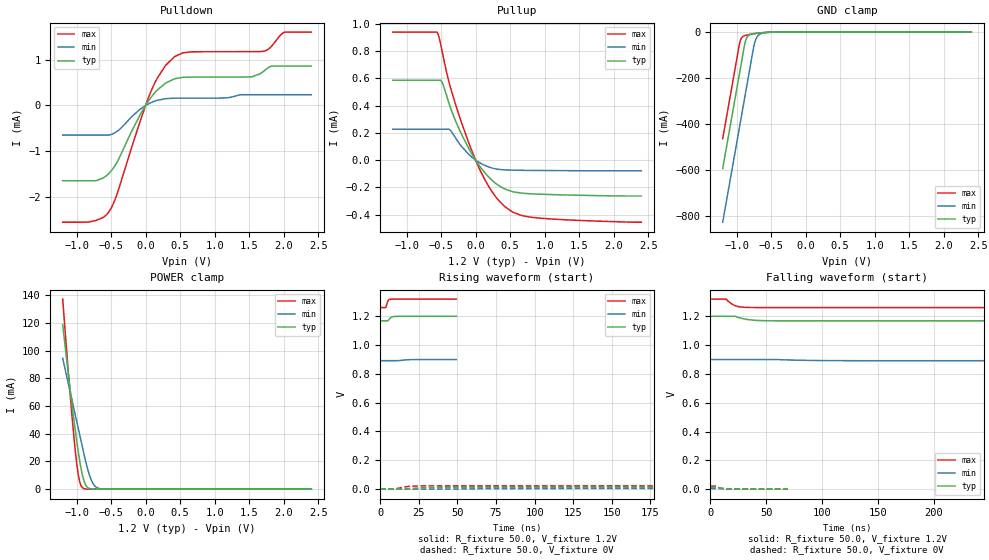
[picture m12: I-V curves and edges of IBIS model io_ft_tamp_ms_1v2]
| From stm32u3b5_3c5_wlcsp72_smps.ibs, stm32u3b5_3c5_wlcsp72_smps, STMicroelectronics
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[Model]   io_ft_tamp_ms_1v2
Model_type I/O
Polarity   Non-Inverting
Enable   Active-Low
| CAP_THRESHOLD on pad IOFT is "UDTCAPC" :
| Rising=30.0% of vddios   Falling=70.0% of vddios
| C_comp min and max val. don't necessarily correlate with the min and max pvt
| but are the smallest and greatest pad capacitance found.
| var   typ   min   max
C_comp   2.39258pF  2.36010pF  2.41953pF
|C_comp_pullup   1.38909pF  1.28768pF  1.47308pF
|C_comp_pulldown   1.00349pF  1.07242pF  946.45422fF
Vinl = 450.0mV
Vinh = 660.0mV
Vmeas = 600.0mV   | Reference voltage for timing measurements
Cref  = 50.0pF   | Timing specification test load capacitance value
Rref  = 1.0MOhm   | Timing specification test load resistance value
Vref  = 660.0mV   | Timing specification test load voltage
[Model Spec]
| TIME_THRESHOLD on pin ZIV11 is "CMOS" :
| Rising=50.0% of vdd   Falling=50.0% of vdd
Vinl 439.50000mV 331.50001mV 485.50000mV
Vinh 752.50000mV 552.50001mV 837.50000mV
| variable   typ   min   max
[Temperature Range] 25.0 130.0 -40.0
| variable   typ   min   max
[Voltage Range] 1.2V 900.0mV 1.32V
| variable   typ   min   max
[POWER Clamp Reference] 1.2V 900.0mV 1.32V
| variable   typ   min   max
[GND Clamp Reference] 0V 0V 0V
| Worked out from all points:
|   slope of the pulldown table from 0 to 0.18 V, typ, clamps not added: 514 ohm
|   slope of the pullup table from 0 to 0.18 V, typ, clamps not added: 1.52 kohm
|   GND clamp passes 1 mA (typ) near -0.53 V on its own axis
|   POWER clamp passes 1 mA (typ) near -0.83 V on its own axis
[POWER Clamp]
-1.2V     118.8mA    94.44mA    137.2mA
-1.09V    71.2mA     69.75mA    67.14mA
-1.02V    43.22mA    54.03mA    28.67mA
-990mV    32.26mA    47.3mA     15.78mA
-970mV    25.49mA    42.81mA    9.257mA
-940mV    16.45mA    36.08mA    3.257mA
-910mV    9.238mA    29.34mA    904.6uA
-860mV    2.387mA    18.53mA    87.46uA
-790mV    204.6uA    7.049mA    3.101uA
-730mV    21.91uA    2.041mA    176.4nA
-660mV    1.594uA    337.6uA    6.258nA
2.4V      0A         0A         0A
[GND Clamp]
-1.2V     -593.4mA   -826.9mA   -463.7mA
-960mV    -185.4mA   -418.9mA   -55.68mA
-940mV    -151.4mA   -384.9mA   -33.02mA
-880mV    -50.24mA   -282.9mA   -15.1mA
-850mV    -23.55mA   -231.9mA   -12.72mA
-810mV    -11.44mA   -163.9mA   -10.41mA
-740mV    -5.957mA   -49.45mA   -7.062mA
-710mV    -4.858mA   -24.97mA   -5.804mA
-670mV    -3.677mA   -10.87mA   -4.301mA
-590mV    -1.88mA    -3mA       -1.97mA
-390mV    -51.73uA   -182.4uA   -18.95uA
2.4V      708.1pA    117.2nA    245.1pA
| variable   typ   min   max
[Pullup Reference] 1.2V 900.0mV 1.32V
| variable   typ   min   max
[Pulldown Reference] 0V 0V 0V
[Pullup]
-1.2V     585.3uA    226.4uA    938.6uA
-550mV    585.3uA    226.4uA    931.1uA
-480mV    564.6uA    226.4uA    788uA
-360mV    379.5uA    215.3uA    526uA
-230mV    218.5uA    117.8uA    314.5uA
-80mV     67.47uA    32.57uA    100.5uA
50mV      -37.39uA   -16.36uA   -57.25uA
170mV     -113.3uA   -46.43uA   -175.6uA
420mV     -211.4uA   -71.81uA   -339.7uA
540mV     -232.4uA   -73.87uA   -382.1uA
790mV     -246.7uA   -75.44uA   -417.9uA
2.4V      -263.1uA   -78.22uA   -455.1uA
[Pulldown]
-1.2V     -1.647mA   -647.6uA   -2.554mA
-730mV    -1.647mA   -647.6uA   -2.52mA
-530mV    -1.485mA   -646.4uA   -2.323mA
-420mV    -1.261mA   -574.4uA   -1.968mA
80mV      177.8uA    62.75uA    313.5uA
290mV     489.8uA    149.3uA    878.6uA
420mV     583.8uA    159.4uA    1.068mA
670mV     620.6uA    160.1uA    1.174mA
1.54V     627.5uA    235.3uA    1.178mA
1.71V     748.6uA    235.3uA    1.186mA
2.01V     861.3uA    235.3uA    1.602mA
2.4V      861.3uA    235.3uA    1.605mA
[Ramp]
dV/dt_r 7.61866mV/11.09128ns 2.27339mV/29.40618ns 13.1246mV/6.32986ns
dV/dt_f 18.65968mV/11.75988ns 4.80655mV/28.97859ns 35.31857mV/7.20532ns
R_load = 50.0
| Removed startup time: 0s 0s 0s  .
| Removed end time: 49.25ns.
[Rising Waveform]
R_fixture   = 50.0
V_fixture   = 1.2V
V_fixture_min = 900.0mV
V_fixture_max = 1.32V
0s        1.169V     892mV      1.261V
3.5ns     1.169V     892mV      1.261V
3.75ns    1.169V     892mV      1.266V
5.05ns    1.171V     892mV      1.308V
5.7ns     1.179V     892mV      1.316V
6.45ns    1.188V     892mV      1.319V
8.05ns    1.197V     892mV      1.32V
10.05ns   1.199V     892mV      1.32V
21.15ns   1.2V       899.4mV    1.32V
49.25ns   1.2V       899.9mV    1.32V
| Removed startup time: 0s 0s 0s  .
| Removed end time: 499.25ns.
[Falling Waveform]
R_fixture   = 50.0
V_fixture   = 1.2V
V_fixture_min = 900.0mV
V_fixture_max = 1.32V
0s        1.2V       900mV      1.32V
14.25ns   1.2V       900mV      1.32V
19.25ns   1.2V       900mV      1.286V
23ns      1.199V     900mV      1.272V
27.65ns   1.187V     900mV      1.265V
34.55ns   1.177V     900mV      1.262V
40.75ns   1.172V     900mV      1.261V
61.15ns   1.169V     899.8mV    1.261V
122.3ns   1.169V     892.3mV    1.261V
499.3ns   1.169V     892mV      1.261V
| Removed startup time: 0s 0s 0s  .
| Removed end time: 249.25ns.
[Rising Waveform]
R_fixture   = 50.0
V_fixture   = 0V
V_fixture_min = 0V
V_fixture_max = 0V
0s        10.41nV    204nV      9.892nV
9.3ns     -257.5uV   791.2nV    -31.07uV
14.95ns   -66.09uV   -91.02uV   13.2mV
18.1ns    2.011mV    -77.4uV    18.03mV
21.35ns   4.747mV    -98.93uV   20.32mV
28.15ns   9.409mV    -43.98uV   21.65mV
35.6ns    11.67mV    -7.941uV   21.84mV
50.9ns    12.6mV     501.7uV    21.86mV
101.8ns   12.69mV    3.541mV    21.87mV
249.3ns   12.7mV     3.789mV    21.87mV
| Removed startup time: 0s 0s 0s  .
| Removed end time: 69.25ns.
[Falling Waveform]
R_fixture   = 50.0
V_fixture   = 0V
V_fixture_min = 0V
V_fixture_max = 0V
0s        12.7mV     3.795mV    21.88mV
4.2ns     12.69mV    3.796mV    21.86mV
5.45ns    12.62mV    3.795mV    17.73mV
9.9ns     7.117mV    3.794mV    5.22mV
12.2ns    4.757mV    3.807mV    1.581mV
14.8ns    2.603mV    3.502mV    400uV
18.4ns    751.2uV    2.904mV    176.9uV
22.65ns   208.5uV    2.258mV    79.86uV
42.45ns   17.9uV     299.2uV    1.022uV
69.25ns   441.6nV    32.17uV    35.27nV
